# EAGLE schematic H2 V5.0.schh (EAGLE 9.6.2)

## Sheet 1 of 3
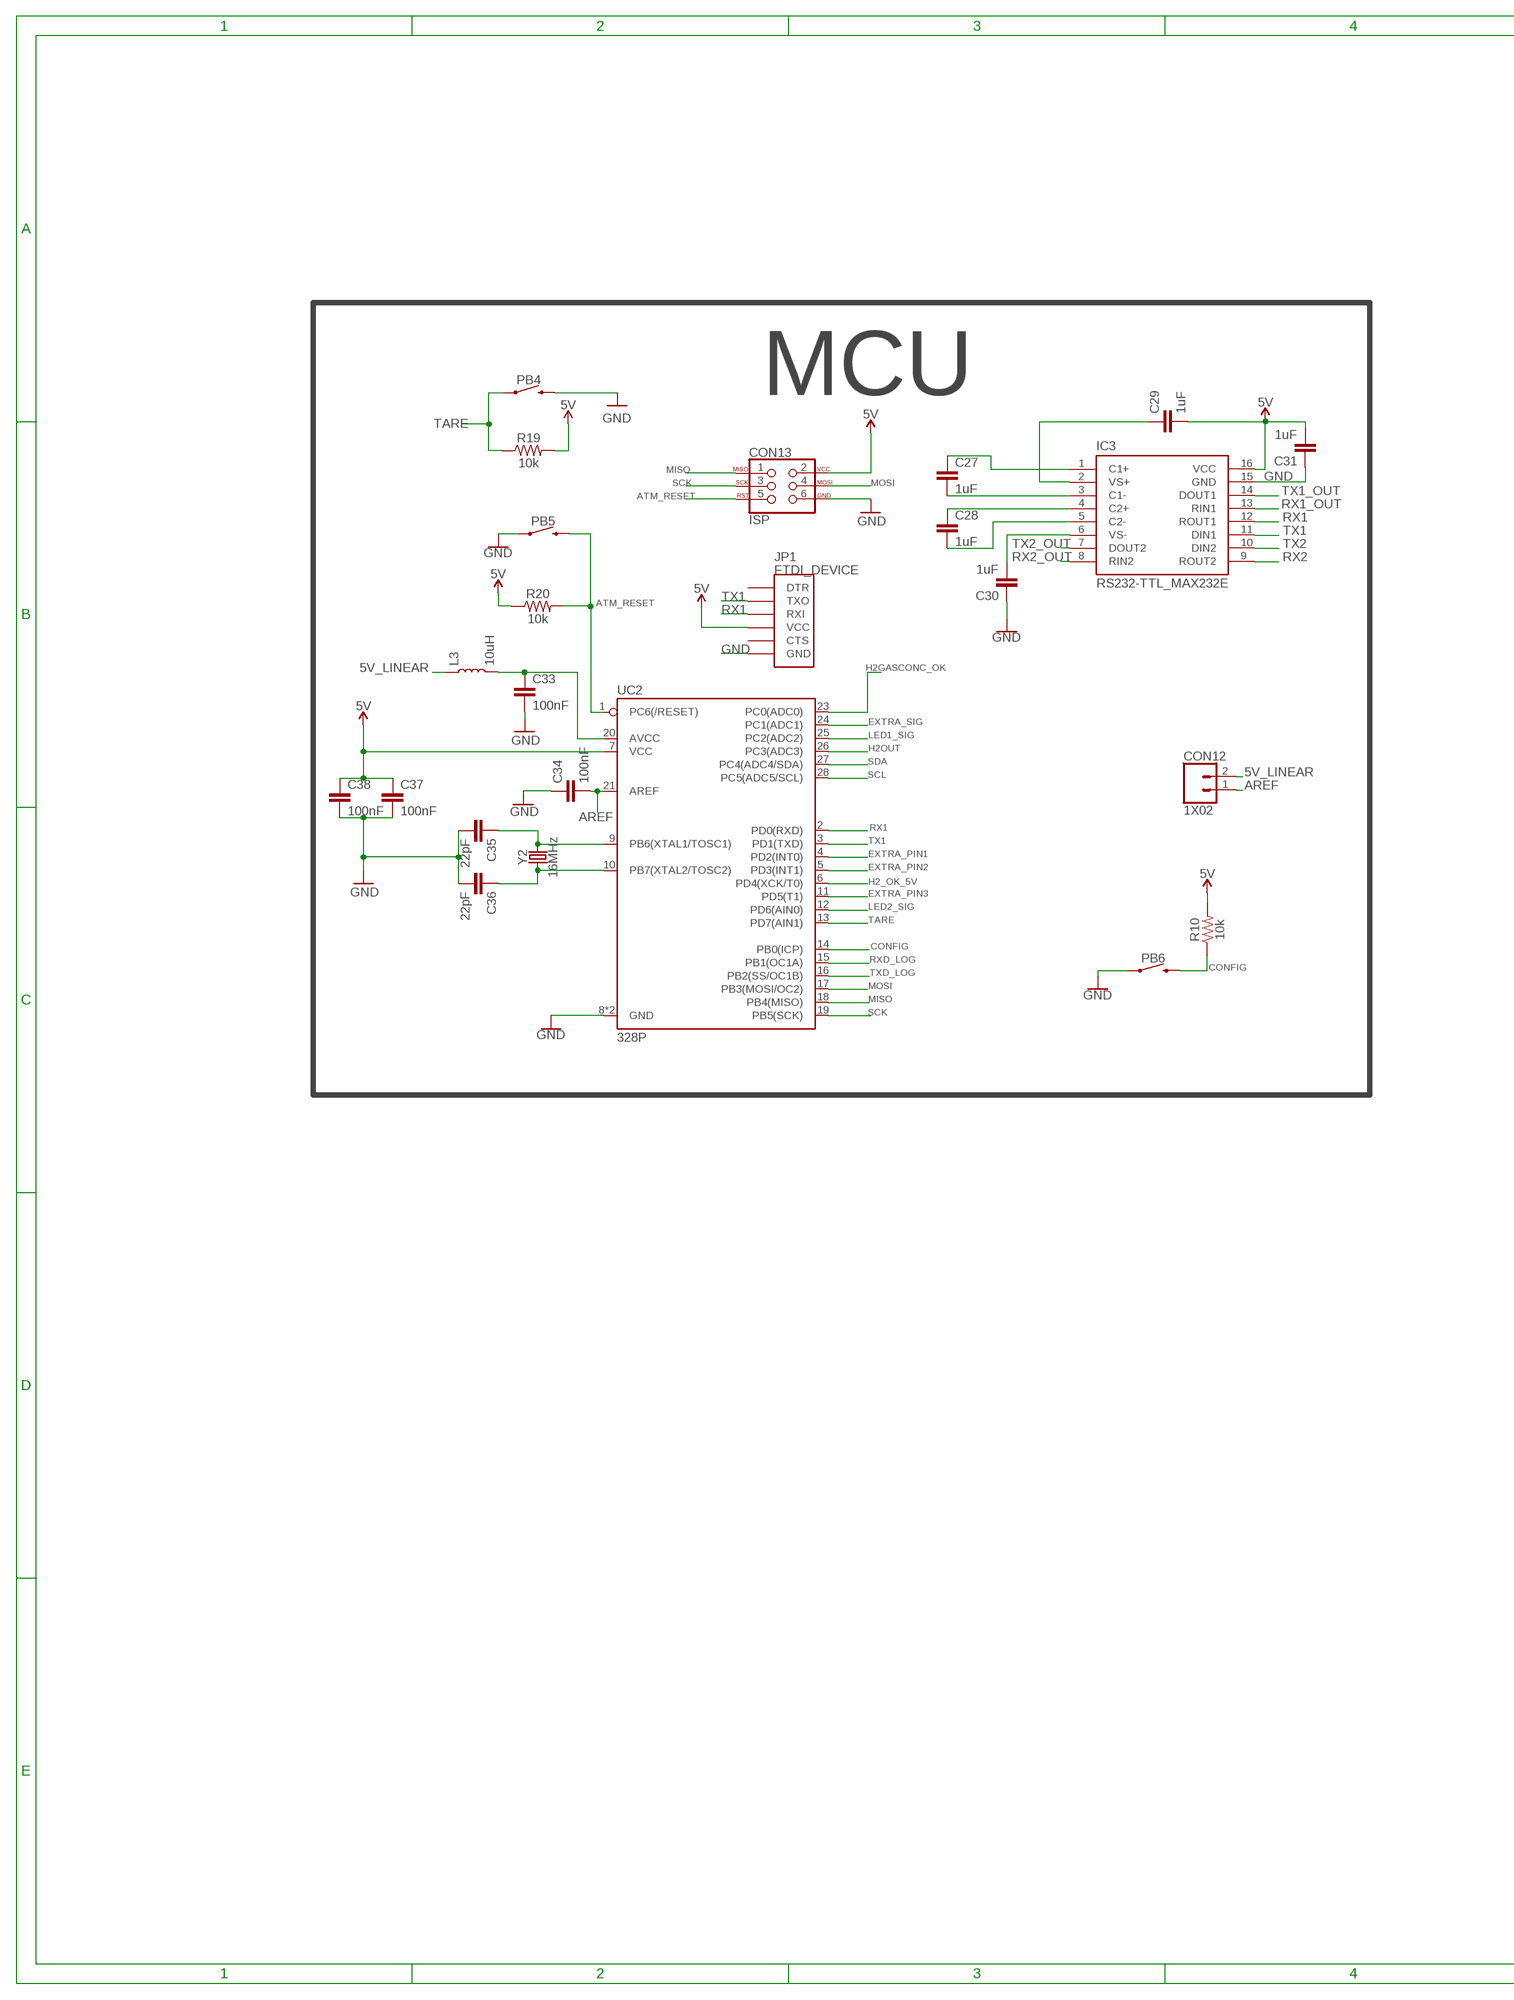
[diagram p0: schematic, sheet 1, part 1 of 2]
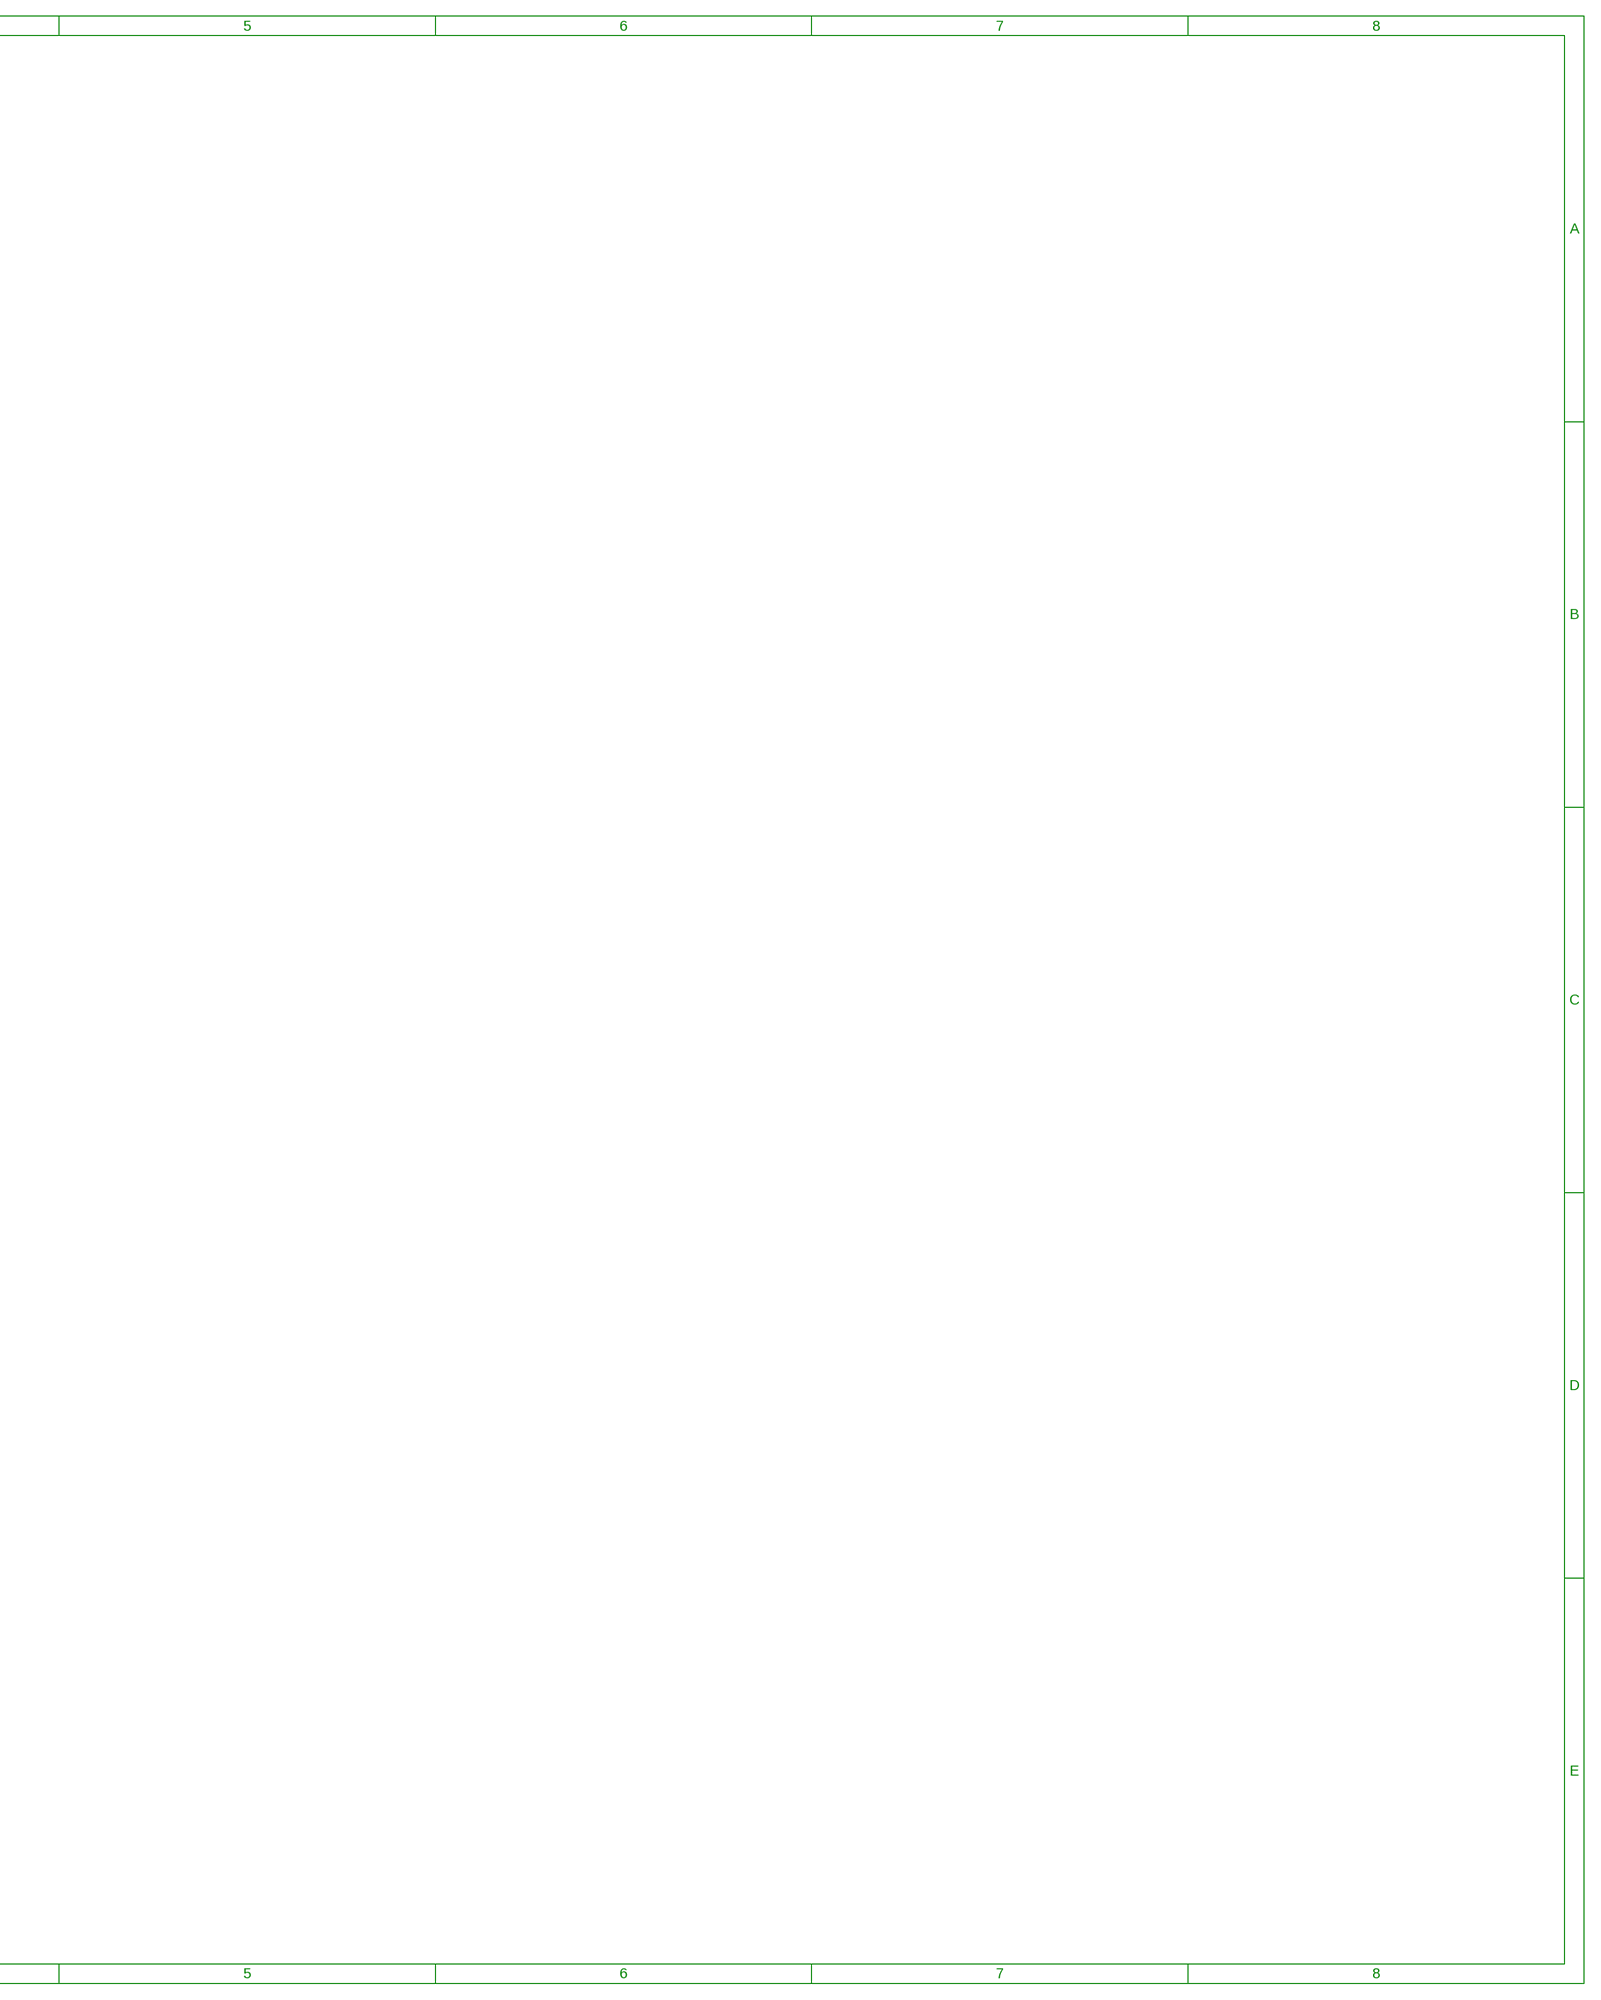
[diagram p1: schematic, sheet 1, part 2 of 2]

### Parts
C27  1uF  CAPACITOR_0805  [0805]
C28  1uF  CAPACITOR_0805  [0805]
C29  1uF  CAPACITOR_0805  [0805]
C30  1uF  CAPACITOR_0805  [0805]
C31  1uF  CAPACITOR_0805  [0805]
C33  100nF  CAPACITOR_0805  [0805]
C34  100nF  CAPACITOR_0805  [0805]
C35  22pF  CAPACITOR_0805  [0805]
C36  22pF  CAPACITOR_0805  [0805]
C37  100nF  CAPACITOR_0805  [0805]
C38  100nF  CAPACITOR_0805  [0805]
CON12  1X02  [1X02]
CON13  ISP  [ISP_CONNECTOR]
IC3  RS232-TTL_MAX232E  [DIP16]
JP1  FTDI_DEVICE  [FTDI_DEVICE_SIDE]
L3  10uH  INDUCTOR_0805  [0805]
PB4  PUSHBUTTON  [PUSHBUTTON]
PB5  PUSHBUTTON  [PUSHBUTTON]
PB6  PUSHBUTTON  [PUSHBUTTON]
R10  10k  RESISTOR_0805  [0805]
R19  10k  RESISTOR_0805  [0805]
R20  10k  RESISTOR_0805  [0805]
UC2  328P  ATMEGA328P_DIP28  [DIP28]
Y2  16MHz  CRYSTAL-16MHZPTH-HC49US  [HC49US]

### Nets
5V: C29.2 C31.2 C37.1 C38.1 CON13.2 IC3.16(VCC) JP1.P$4(VCC) R10.2 R19.2 R20.1 UC2.7(VCC) ; also sheet 2,3
5V_LINEAR: CON12.2 L3.1 ; also sheet 2,3
AREF: C34.2 CON12.1 UC2.21(AREF)
ATM_RESET: CON13.5 PB5.3 PB5.4 R20.2 UC2.1(PC6(/RESET))
CONFIG: PB6.3 PB6.4 R10.1 UC2.14(PB0(ICP))
EXTRA_PIN1: UC2.4(PD2(INT0)) ; also sheet 3
EXTRA_PIN2: UC2.5(PD3(INT1)) ; also sheet 3
EXTRA_PIN3: UC2.11(PD5(T1)) ; also sheet 3
EXTRA_SIG: UC2.24(PC1(ADC1)) ; also sheet 3
GND: C30.1 C31.1 C33.2 C34.1 C35.2 C36.2 C37.2 C38.2 CON13.6 IC3.15(GND) JP1.P$6(GND) PB4.3 PB4.4 PB5.1 PB5.2 PB6.1 PB6.2 UC2.8(GND) UC2.22(GND) ; also sheet 2,3
H2_OK_5V: UC2.6(PD4(XCK/T0)) ; also sheet 3
H2GASCONC_OK: UC2.23(PC0(ADC0)) ; also sheet 3
H2OUT: UC2.26(PC3(ADC3)) ; also sheet 2
LED1_SIG: UC2.25(PC2(ADC2)) ; also sheet 2
LED2_SIG: UC2.12(PD6(AIN0)) ; also sheet 2
MISO: CON13.1 UC2.18(PB4(MISO))
MOSI: CON13.4 UC2.17(PB3(MOSI/OC2))
N$14: C35.1 UC2.9(PB6(XTAL1/TOSC1)) Y2.2
N$17: C36.1 UC2.10(PB7(XTAL2/TOSC2)) Y2.1
N$19: C33.1 L3.2 UC2.20(AVCC)
N$24: C27.2 IC3.3(C1-)
N$26: C27.1 IC3.1(C1+)
N$27: C28.1 IC3.4(C2+)
N$28: C28.2 IC3.5(C2-)
N$29: C30.2 IC3.6(VS-)
N$30: C29.1 IC3.2(VS+)
RX1: IC3.12(ROUT1) JP1.P$3(RXI) UC2.2(PD0(RXD)) ; also sheet 3
RX1_OUT: IC3.13(RIN1) ; also sheet 3
RX2: IC3.9(ROUT2) ; also sheet 3
RX2_OUT: IC3.8(RIN2) ; also sheet 3
RXD_LOG: UC2.15(PB1(OC1A)) ; also sheet 2
SCK: CON13.3 UC2.19(PB5(SCK))
SCL: UC2.28(PC5(ADC5/SCL)) ; also sheet 2
SDA: UC2.27(PC4(ADC4/SDA)) ; also sheet 2
TARE: PB4.1 PB4.2 R19.1 UC2.13(PD7(AIN1))
TX1: IC3.11(DIN1) JP1.P$2(TXO) UC2.3(PD1(TXD)) ; also sheet 3
TX1_OUT: IC3.14(DOUT1) ; also sheet 3
TX2: IC3.10(DIN2) ; also sheet 3
TX2_OUT: IC3.7(DOUT2) ; also sheet 3
TXD_LOG: UC2.16(PB2(SS/OC1B)) ; also sheet 2
Unconnected: JP1.P$1(DTR) JP1.P$5(CTS)

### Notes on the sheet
- MCU

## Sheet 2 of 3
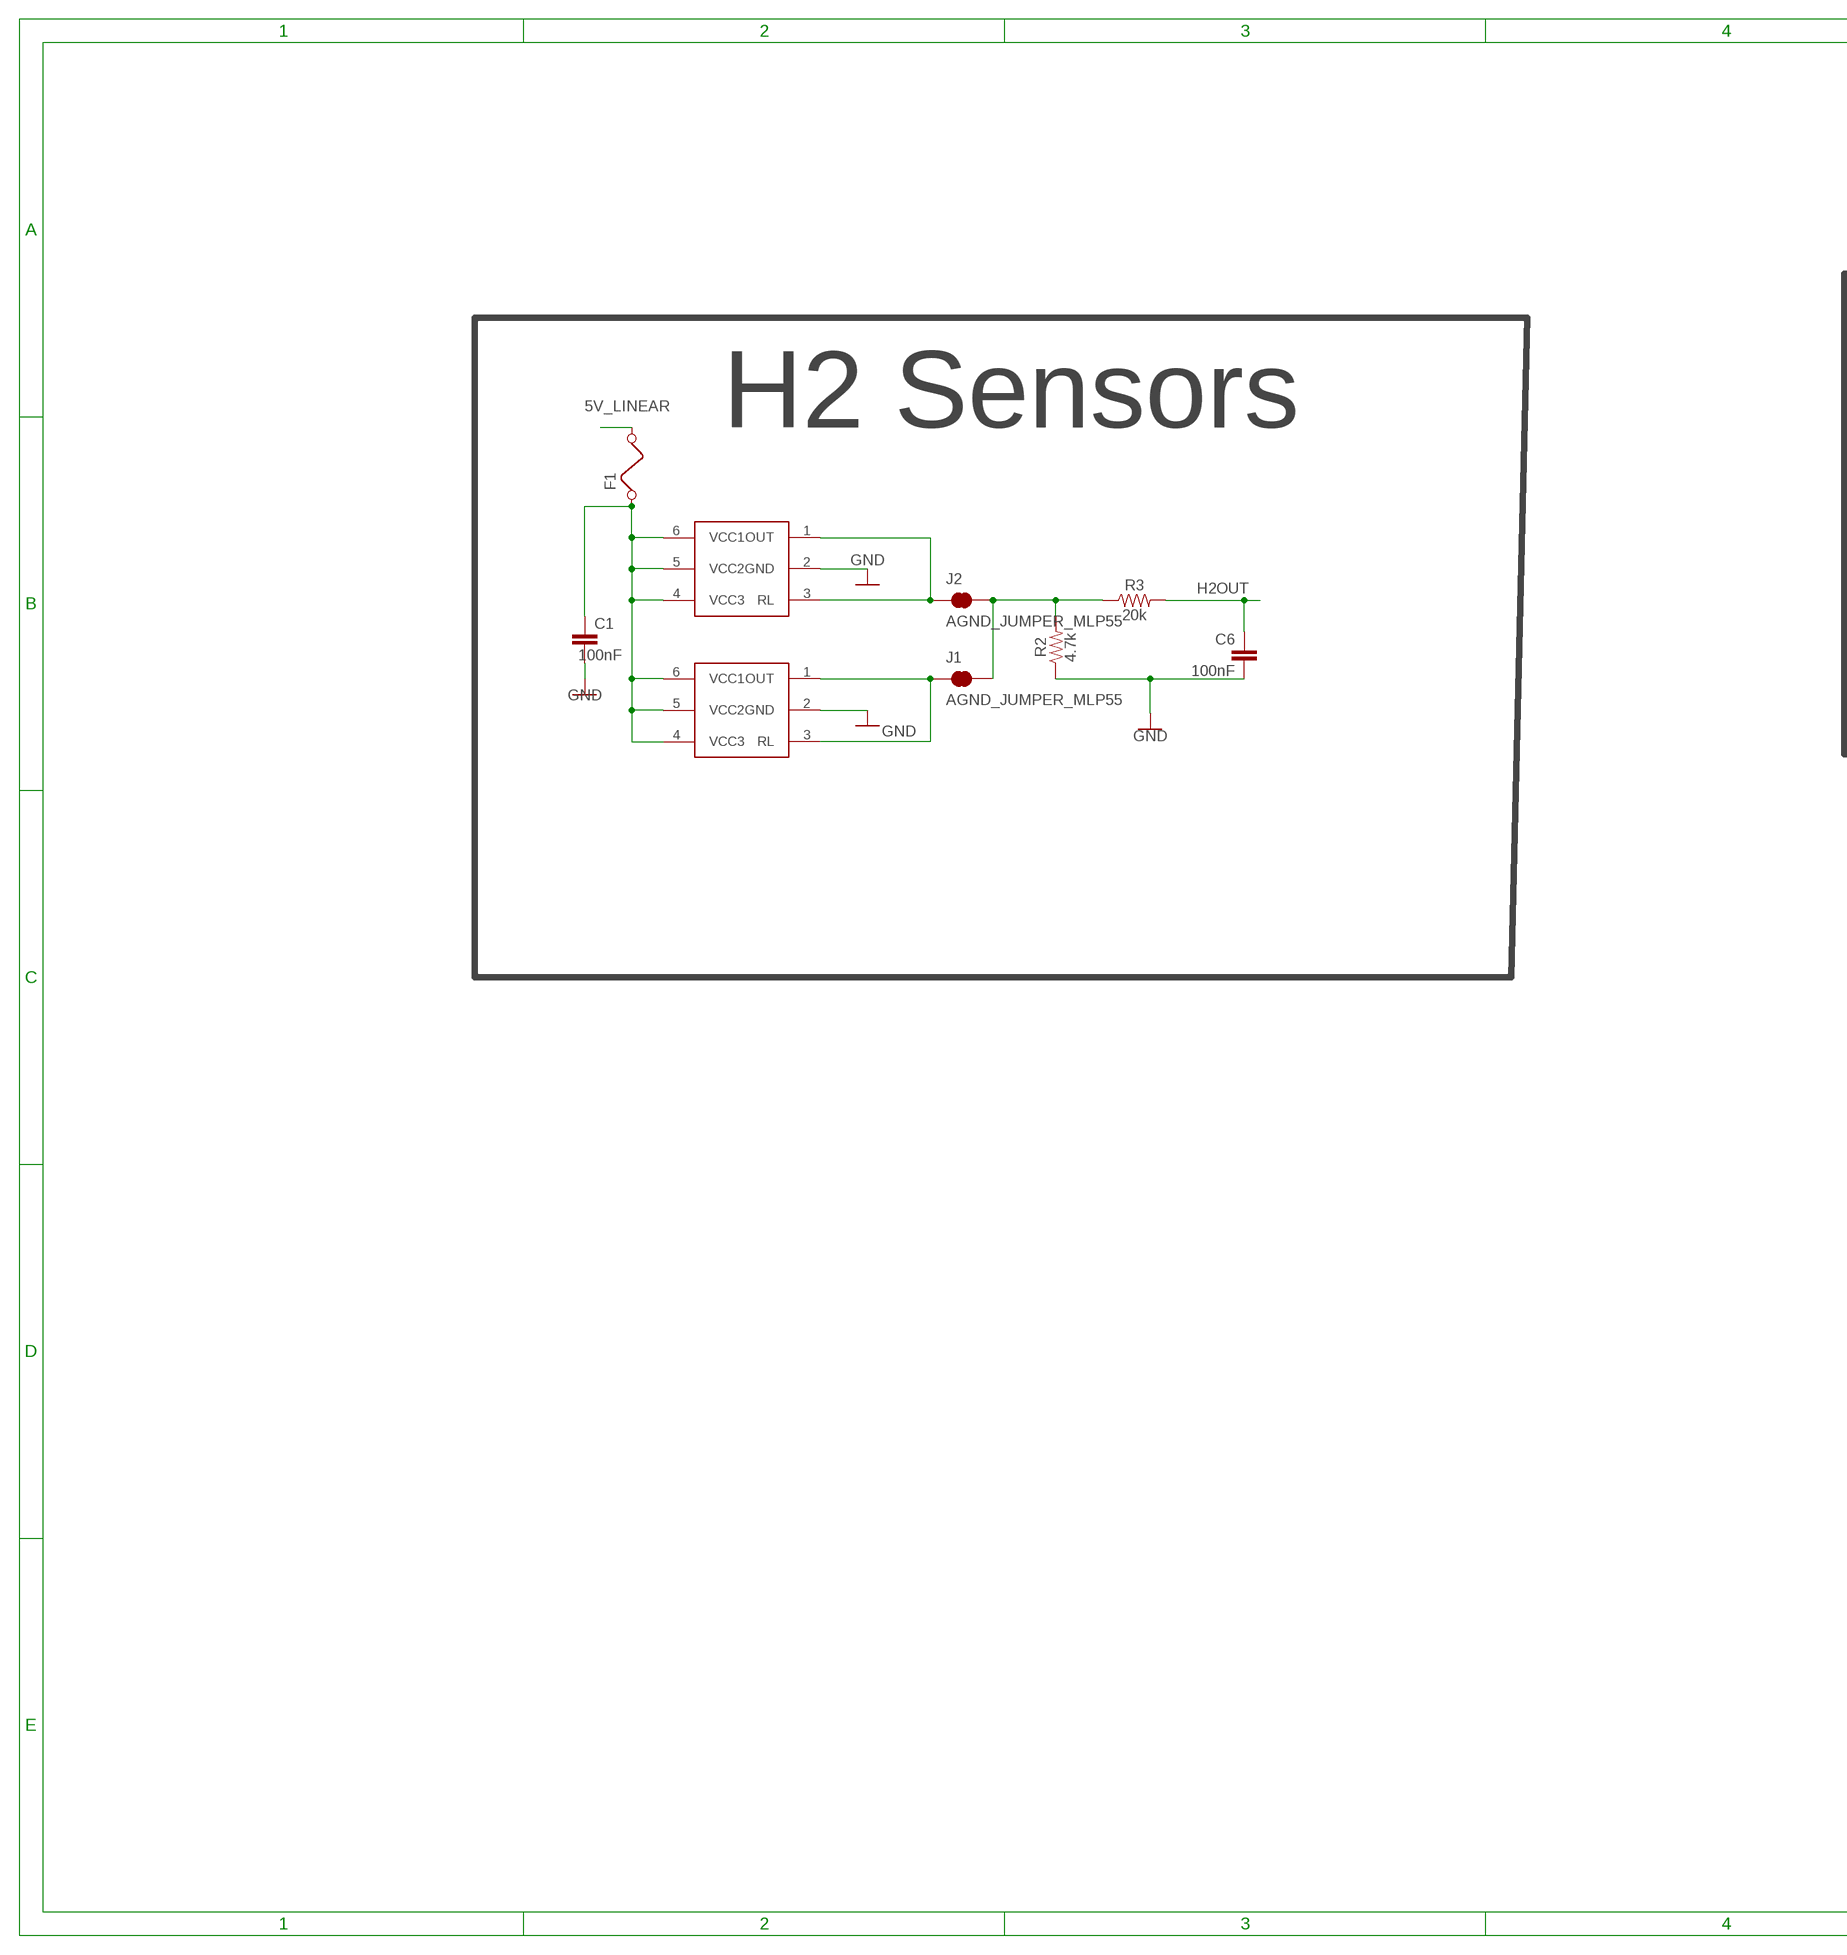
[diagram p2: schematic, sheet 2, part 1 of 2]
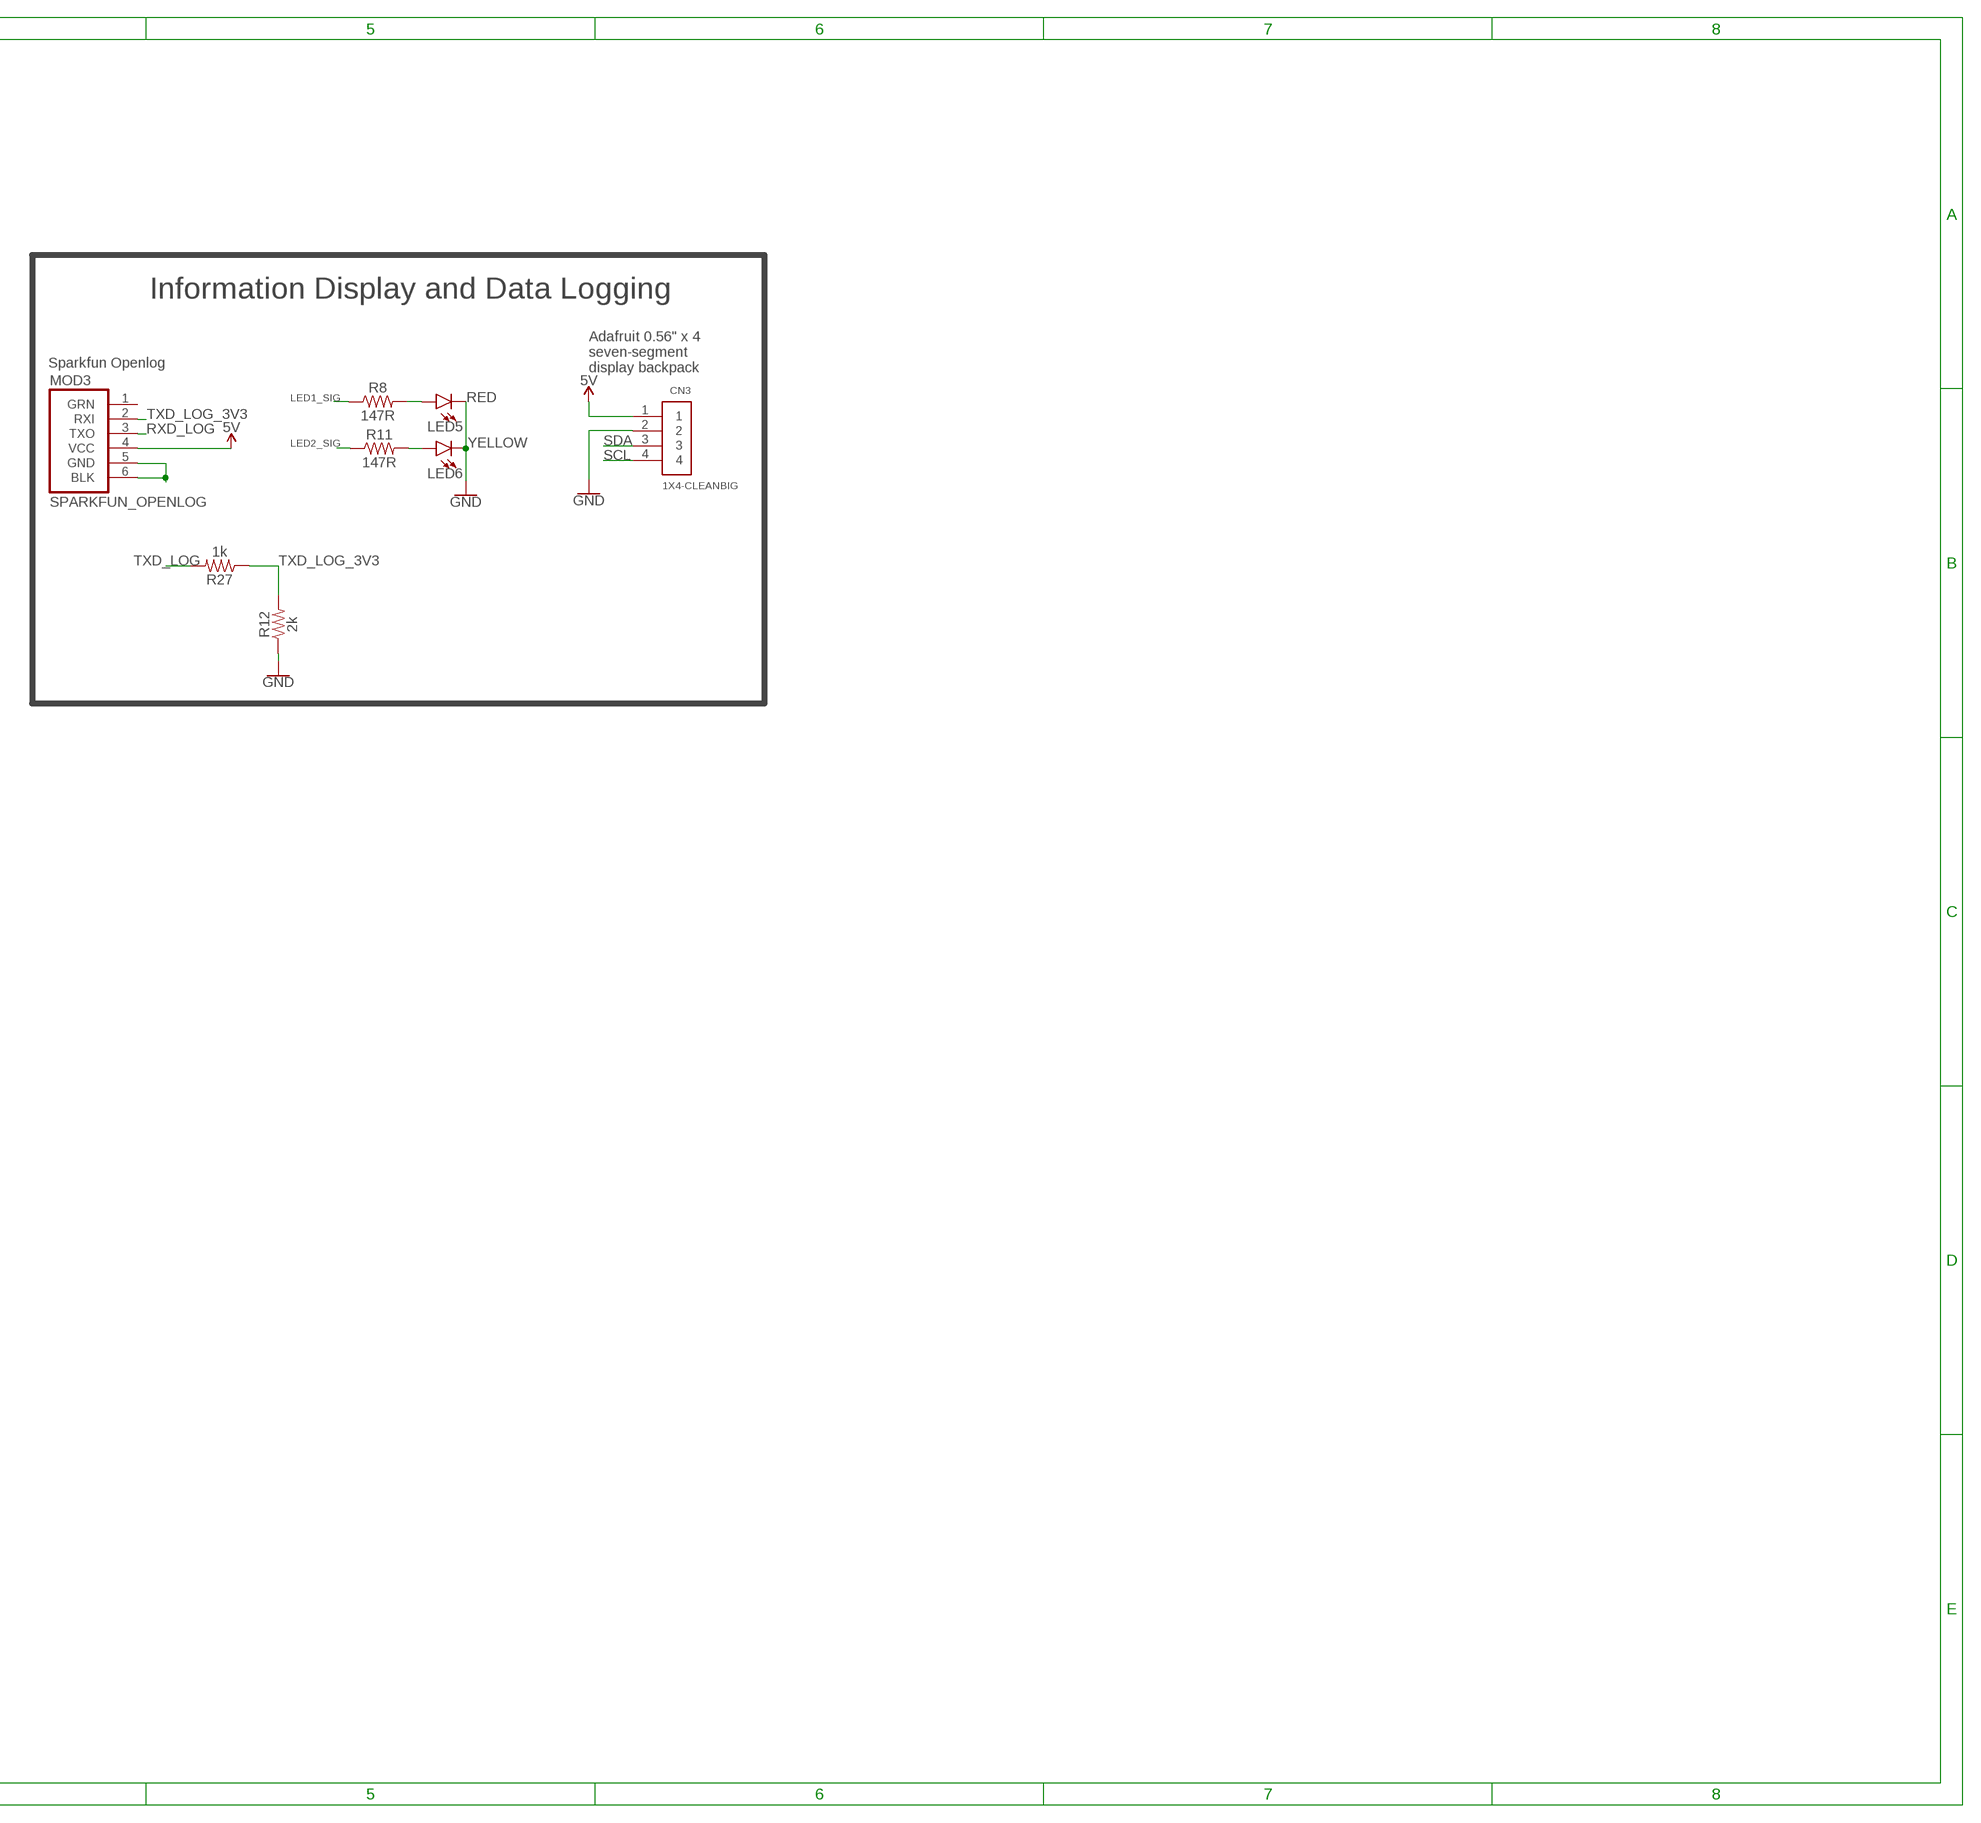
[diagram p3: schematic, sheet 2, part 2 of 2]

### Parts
C1  100nF  CAPACITOR_0805  [0805]
C6  100nF  CAPACITOR_0805  [0805]
CN3  1X4-CLEANBIG  [1X04-CLEANBIG]
F1  FUSE_1210  [1210]
J1  AGND_JUMPER_MLP55  [AGND_JUMPER_MLP55]
J2  AGND_JUMPER_MLP55  [AGND_JUMPER_MLP55]
LED5  RED  LED_0805  [0805_LED]
LED6  YELLOW  LED_0805  [0805_LED]
MOD3  SPARKFUN_OPENLOG  [SPARKFUN_OPENLOG]
R2  4.7k  RESISTOR_0805  [0805]
R3  20k  RESISTOR_0805  [0805]
R8  147R  RESISTOR_0805  [0805]
R11  147R  RESISTOR_0805  [0805]
R12  2k  RESISTOR_0805  [0805]
R27  1k  RESISTOR_0805  [0805]
U$1  MQ-8MQ-8  [MQ-8]
U$2  MQ-8MQ-8  [MQ-8]

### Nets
5V: CN3.1 MOD3.4(VCC) ; also sheet 1,3
5V_LINEAR: C1.1 F1.1 F1.2 U$1.4(VCC3) U$1.5(VCC2) U$1.6(VCC1) U$2.4(VCC3) U$2.5(VCC2) U$2.6(VCC1) ; also sheet 1,3
GND: C1.2 C6.2 CN3.2 LED5.2(C) LED6.2(C) R2.1 R12.1 U$1.2(GND) U$2.2(GND) ; also sheet 1,3
H2OUT: C6.1 R3.2 ; also sheet 1
LED1_SIG: R8.1 ; also sheet 1
LED2_SIG: R11.1 ; also sheet 1
N$1: LED5.1(A) R8.2
N$3: J1.P$2 J2.P$2 R2.2 R3.1
N$4: J1.P$1 U$2.1(OUT) U$2.3(RL)
N$6: J2.P$1 U$1.1(OUT) U$1.3(RL)
N$15: LED6.1(A) R11.2
N$16: MOD3.5(GND) MOD3.6(BLK)
RXD_LOG: MOD3.3(TXO) ; also sheet 1
SCL: CN3.4 ; also sheet 1
SDA: CN3.3 ; also sheet 1
TXD_LOG: R27.2 ; also sheet 1
TXD_LOG_3V3: MOD3.2(RXI) R12.2 R27.1
Unconnected: MOD3.1(GRN)

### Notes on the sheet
- Information Display and Data Logging
- Sparkfun Openlog
- Adafruit 0.56" x 4 
  seven-segment 
  display backpack
- H2 Sensors

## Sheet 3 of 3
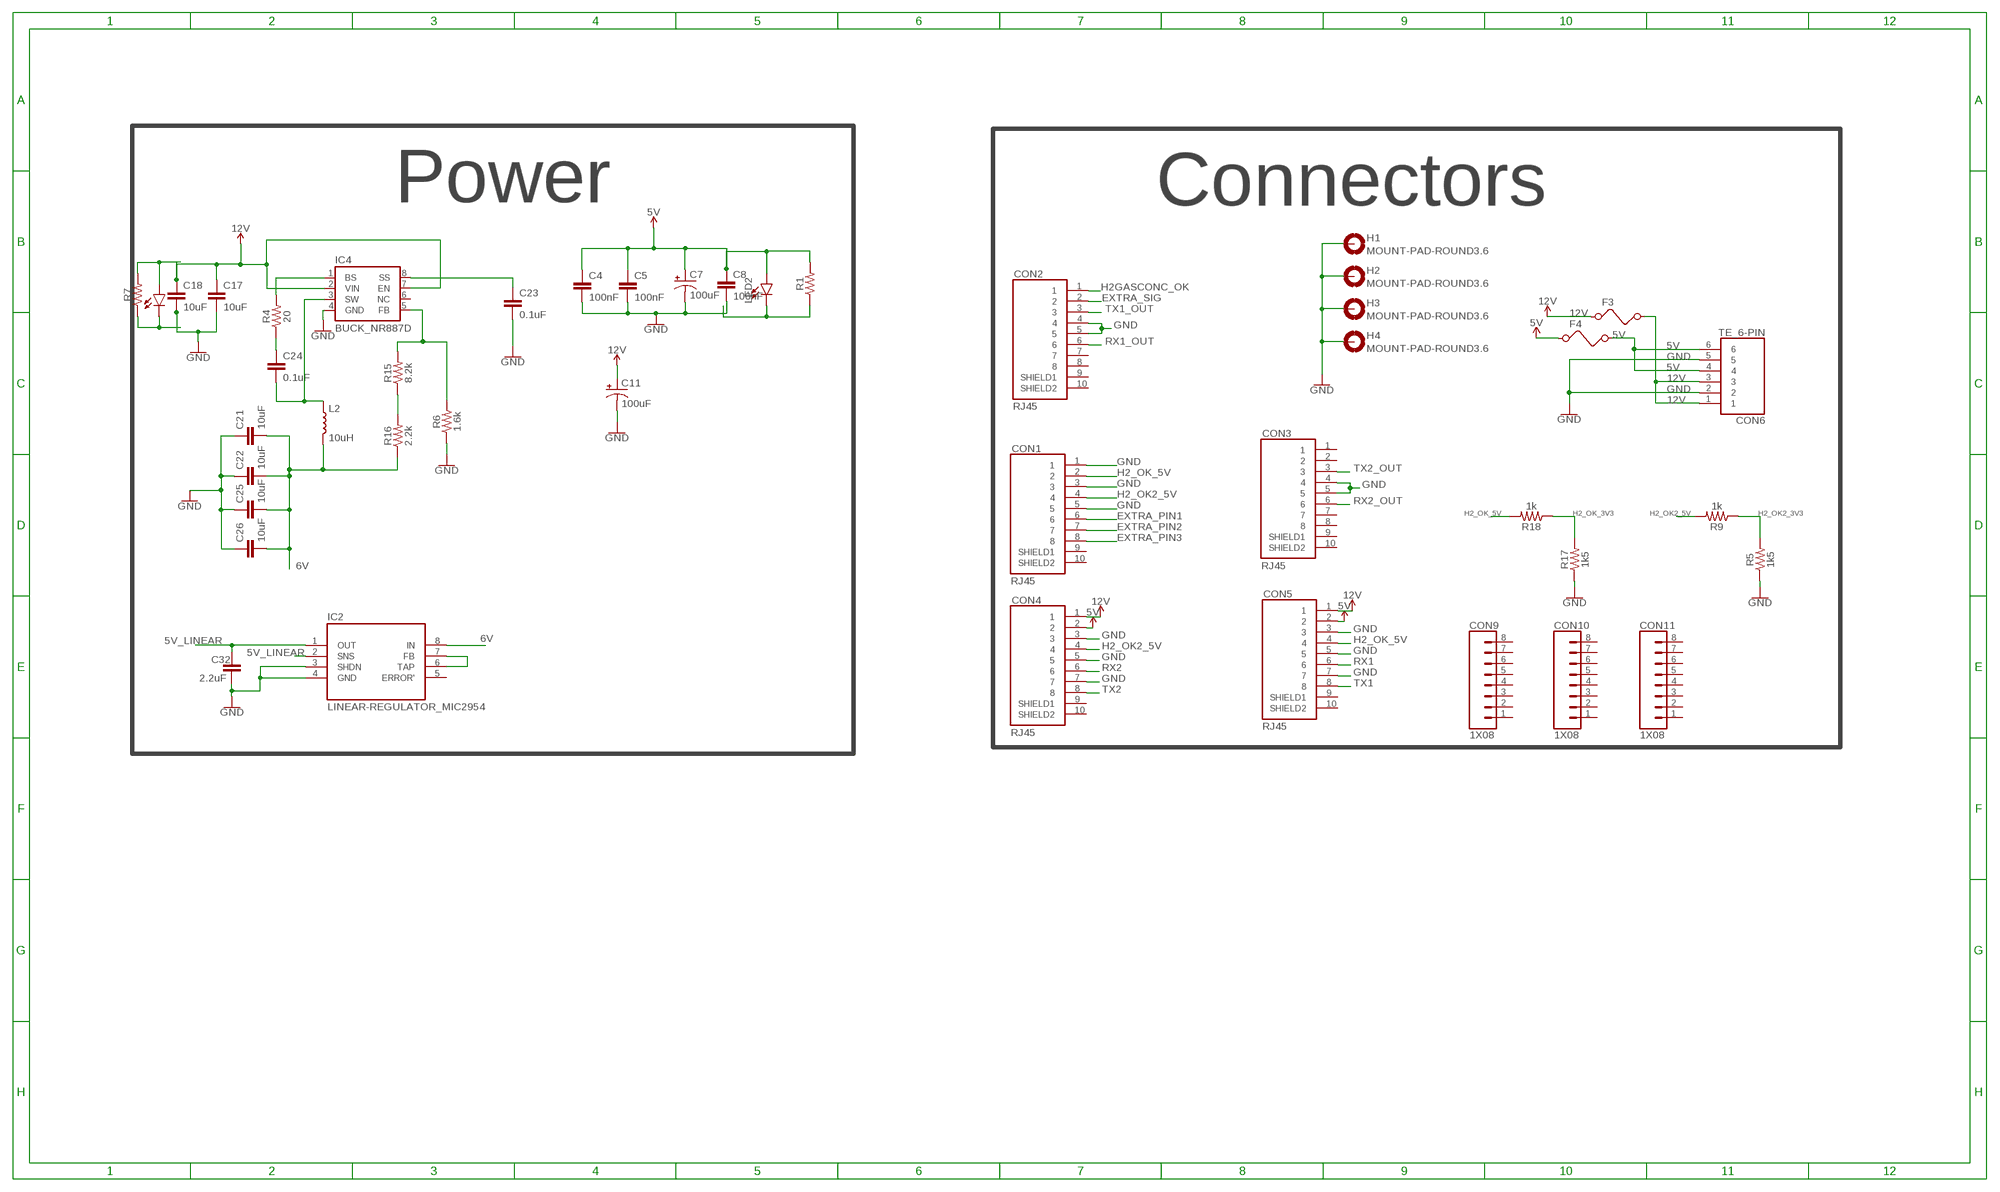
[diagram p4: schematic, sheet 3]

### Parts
C4  100nF  CAPACITOR_0805  [0805]
C5  100nF  CAPACITOR_0805  [0805]
C7  100uF  CAPACITOR_ELECTROLYTIC_100UF  [CAPACITOR_100UF_50V]
C8  100nF  CAPACITOR_0805  [0805]
C11  100uF  CAPACITOR_ELECTROLYTIC_100UF  [CAPACITOR_100UF_50V]
C17  10uF  CAPACITOR_0805  [0805]
C18  10uF  CAPACITOR_0805  [0805]
C21  10uF  CAPACITOR_1210  [1210]
C22  10uF  CAPACITOR_1210  [1210]
C23  0.1uF  CAPACITOR_0805  [0805]
C24  0.1uF  CAPACITOR_0805  [0805]
C25  10uF  CAPACITOR_1210  [1210]
C26  10uF  CAPACITOR_1210  [1210]
C32  2.2uF  CAPACITOR_0805  [0805]
CON1  RJ45  [RJ45]
CON2  RJ45  [RJ45]
CON3  RJ45  [RJ45]
CON4  RJ45  [RJ45]
CON5  RJ45  [RJ45]
CON6  TE_6-PIN  [TE_6-PIN]
CON9  1X08  [1X08]
CON10  1X08  [1X08]
CON11  1X08  [1X08]
F3  FUSE_1210  [1210]
F4  FUSE_1210  [1210]
H1  MOUNT-PAD-ROUND3.6  [3,6-PAD]
H2  MOUNT-PAD-ROUND3.6  [3,6-PAD]
H3  MOUNT-PAD-ROUND3.6  [3,6-PAD]
H4  MOUNT-PAD-ROUND3.6  [3,6-PAD]
IC2  LINEAR-REGULATOR_MIC2954  [SOIC8]
IC4  BUCK_NR887D  [DIP08]
L2  10uH  INDUCTOR_MURATA_DEM8030C  [INDUCTOR_MURATA_DEM8030C]
LED1  LED_0805  [0805_LED]
LED2  LED_0805  [0805_LED]
R1  RESISTOR_0805  [0805]
R4  20  RESISTOR_0805  [0805]
R5  1k5  RESISTOR_0805  [0805]
R6  1.6k  RESISTOR_0805  [0805]
R7  RESISTOR_0805  [0805]
R9  1k  RESISTOR_0805  [0805]
R15  8.2k  RESISTOR_0805  [0805]
R16  2.2k  RESISTOR_0805  [0805]
R17  1k5  RESISTOR_0805  [0805]
R18  1k  RESISTOR_0805  [0805]

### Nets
5V: C4.1 C5.1 C7.+ C8.1 CON4.2 CON5.2 CON6.4 CON6.6 F4.1 F4.2 LED2.1(A) R1.2 ; also sheet 1,2
5V_LINEAR: C32.1 IC2.1(OUT) IC2.2(SNS) ; also sheet 1,2
6V: C21.2 C22.2 C25.2 C26.2 IC2.8(IN) L2.P$2 R16.1
12V: C11.+ C17.1 C18.1 CON4.1 CON5.1 CON6.1 CON6.3 F3.1 F3.2 IC4.2(VIN) IC4.7(EN)
EXTRA_PIN1: CON1.6 ; also sheet 1
EXTRA_PIN2: CON1.7 ; also sheet 1
EXTRA_PIN3: CON1.8 ; also sheet 1
EXTRA_SIG: CON2.2 ; also sheet 1
GND: C4.2 C5.2 C7.- C8.2 C11.- C17.2 C18.2 C21.1 C22.1 C23.2 C25.1 C26.1 C32.2 CON1.1 CON1.3 CON1.5 CON2.4 CON2.5 CON3.4 CON3.5 CON4.3 CON4.5 CON4.7 CON5.3 CON5.5 CON5.7 CON6.2 CON6.5 H1.B3,6(MOUNT) H2.B3,6(MOUNT) H3.B3,6(MOUNT) H4.B3,6(MOUNT) IC2.3(SHDN) IC2.4(GND) IC4.4(GND) R5.1 R6.1 R17.1 ; also sheet 1,2
H2_OK2_3V3: R5.2 R9.1
H2_OK2_5V: CON1.4 CON4.4 R9.2
H2_OK_3V3: R17.2 R18.1
H2_OK_5V: CON1.2 CON5.4 R18.2 ; also sheet 1
H2GASCONC_OK: CON2.1 ; also sheet 1
N$2: C23.1 IC4.8(SS)
N$5: IC4.1(BS) R4.2
N$8: C24.1 R4.1
N$9: C24.2 IC4.3(SW) L2.P$1
N$10: IC4.5(FB) R6.2 R15.2
N$11: IC2.6(TAP) IC2.7(FB)
N$12: LED1.1(A) R7.2
N$13: R15.1 R16.2
N$18: LED2.2(C) R1.1
N$20: LED1.2(C) R7.1
RX1: CON5.6 ; also sheet 1
RX1_OUT: CON2.6 ; also sheet 1
RX2: CON4.6 ; also sheet 1
RX2_OUT: CON3.6 ; also sheet 1
TX1: CON5.8 ; also sheet 1
TX1_OUT: CON2.3 ; also sheet 1
TX2: CON4.8 ; also sheet 1
TX2_OUT: CON3.3 ; also sheet 1
Unconnected: CON1.9(SHIELD1) CON1.10(SHIELD2) CON2.7 CON2.8 CON2.9(SHIELD1) CON2.10(SHIELD2) CON3.1 CON3.2 CON3.7 CON3.8 CON3.9(SHIELD1) CON3.10(SHIELD2) CON4.9(SHIELD1) CON4.10(SHIELD2) CON5.9(SHIELD1) CON5.10(SHIELD2) CON9.1 CON9.2 CON9.3 CON9.4 CON9.5 CON9.6 CON9.7 CON9.8 CON10.1 CON10.2 CON10.3 CON10.4 CON10.5 CON10.6 CON10.7 CON10.8 CON11.1 CON11.2 CON11.3 CON11.4 CON11.5 CON11.6 CON11.7 CON11.8 IC2.5(ERROR') IC4.6(NC)

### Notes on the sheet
- Power | Connectors

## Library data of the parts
C1 C4-C6 C8 C17 C18 C23 C24 C27-C38 = EcoCar-Passives:CAPACITOR_0805
C7 C11 = EcoCar-Passives:CAPACITOR_ELECTROLYTIC_100UF: 50V 100uF Electrolytic Capacitor
C21 C22 C25 C26 = EcoCar-Passives:CAPACITOR_1210
CN3 = adafruit:1X4: 4-pin connector
CON1-CON5 = EcoCar-Connectors:RJ45: RJ45 Connector - Use for signals and low power connections Unshielded Part Number: RJHSE-5080 Unshielded Digikey Part Number: RJHSE-5080-ND Shielded Part Number: RJHSE5E80 Shielded Digikey Part Number: RJHSE5E80-ND
CON6 = EcoCar-Connectors:TE_6-PIN: 6 Pin TE Mini-Universal MATE-N-LOK Part Number: 1-770969-0 Digikey Part Number: A32475-ND Matching Plug: A97674-ND Matching Crimps: A100828CT-ND
CON9-CON11 = EcoCar-Connectors-2.54mm:1X08: 2.54mm (0.1") Header
CON12 = EcoCar-Connectors-2.54mm:1X02: 2.54mm (0.1") Header
CON13 = EcoCar-Microcontrollers:ISP: ISP Header Use for programming microcontrollers such as the 328P
F1 F3 F4 = EcoCar-Fuses-Protection:FUSE_1210: 1210 Surface Mount Fuse
H1-H4 = holes:MOUNT-PAD-ROUND: MOUNTING PAD, round
IC2 = EcoCar-Integrated-Circuits:LINEAR-REGULATOR_MIC2954: 5V/Adjustable 250mA Low-Dropout Linear Regulator Manufacturer: Microchip Part Number: MIC2954-08YM-TR Digikey Part Number: 576-1156-1-ND
IC3 = EcoCar-Integrated-Circuits:RS232-TTL_MAX232E: Dual 5V TTL to RS-232 Converter Manufacturer: Texas Instruments Part Number: MAX232EIN Digikey Part Number: 296-27963-5-ND
IC4 = EcoCar-Integrated-Circuits:BUCK_NR887D: Sanken 2A Buck Converter Manufacturer: Sanken Part Number: NR887D Digikey Part Number: NR887D-ND
J1 J2 = EcoCar-Miscellaneous:AGND_JUMPER_MLP55
JP1 = SparkFun-Connectors:FTDI_DEVICE: Connector which mates to FTDI basic or FTDI cable.
L2 = EcoCar-Passives:INDUCTOR_MURATA_DEM8030C: Murata DEM8030C Series Inductor
L3 = EcoCar-Passives:INDUCTOR_0805
LED1 LED2 LED5 LED6 = EcoCar-Discrete-Semiconductors:LED_0805
MOD3 = EcoCar-Modules:SPARKFUN_OPENLOG: Sparkfun Openlog Manufacturer: Sparkfun Part Number: DEV-13712 Digikey Part Number: 1568-1368-ND
PB4-PB6 = EcoCar-Electromechanical:PUSHBUTTON: Pushbutton
R1-R12 R15-R20 R27 = EcoCar-Passives:RESISTOR_0805
U$1 U$2 = donny_library:MQ-8
UC2 = EcoCar-Microcontrollers:ATMEGA328P_DIP28: ATmega328P Manufacturer: Microchip Part Number: ATMEGA328P-PU Digikey Part Number: ATMEGA328P-PU-ND; PROD_ID: IC-09136
Y2 = EcoCar-Microcontrollers:CRYSTAL-16MHZ: 16MHz Crystal Oscillator; PROD_ID: XTAL-08181; SF_ID: COM-00536

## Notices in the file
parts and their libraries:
SparkFun: Licensing: CC v3.0 Share-Alike You are welcome to use this library for commercial purposes.
SparkFun-Connectors: Licensing: Creative Commons ShareAlike 4.0 International - https://creativecommons.org/licenses/by-sa/4.0
